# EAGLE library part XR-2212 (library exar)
Precision PHASE-LOCKED LOOP
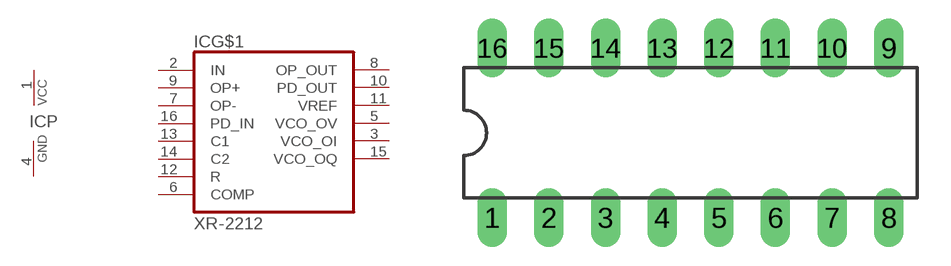
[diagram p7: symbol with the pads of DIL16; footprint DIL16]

Designator prefix IC; gates G$1=XR-2212 P=PWRN

## XR-2212 (OC_FARNELL: unknown; OC_NEWARK: unknown)  [DIL16]
1  P:VCC  pwr
2  G$1:IN  in
3  G$1:VCO_OI  out
4  P:GND  pwr
5  G$1:VCO_OV  out
6  G$1:COMP  in
7  G$1:OP-  in
8  G$1:OP_OUT  out
9  G$1:OP+  in
10  G$1:PD_OUT  out
11  G$1:VREF  out
12  G$1:R  in
13  G$1:C1  in
14  G$1:C2  in
15  G$1:VCO_OQ  out
16  G$1:PD_IN  in

## Footprint DIL16 (pad centres in mm)
Dual In Line Package
drill 0.813 long: 1 -8.89,-3.81; 2 -6.35,-3.81; 3 -3.81,-3.81; 4 -1.27,-3.81; 5 1.27,-3.81; 6 3.81,-3.81; 7 6.35,-3.81; 8 8.89,-3.81; 9 8.89,3.81; 10 6.35,3.81; 11 3.81,3.81; 12 1.27,3.81; 13 -1.27,3.81; 14 -3.81,3.81; 15 -6.35,3.81; 16 -8.89,3.81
